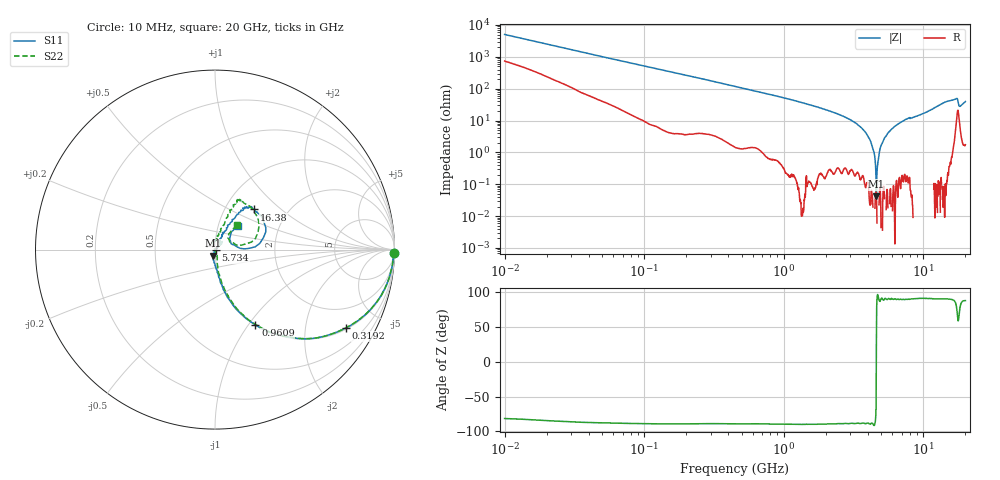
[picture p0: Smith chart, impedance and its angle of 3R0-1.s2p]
!Keysight Technologies,P5008B,MY61100088,A.16.20.02
!Date: Monday, May 27, 2024 14:41:35
!Correction: S11(C* 2-Port  )
!S21(C* 2-Port  )
!S12(C* 2-Port  )
!S22(C* 2-Port  )
!S2P File: Measurements: S11, S21, S12, S22:Log Frequency Sweep
# Hz S  dB  R 50
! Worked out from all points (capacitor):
!   1601 points, 10 MHz to 20 GHz, reference 50 ohm
!   read as one part in series: C = 3.2 pF near 10.39 MHz
!   lowest |Z| = 41.9 mohm at 4.608 GHz (marker M1)
!   series resonance near 4.605 GHz, so ESL is about 370 pH
!   S11 on the Smith chart (normalised r, x): 10 MHz: open; 319.2 MHz: 1.05, -3.30; 960.9 MHz: 1.00, -1.08; 5.734 GHz: 1.01, -0.00; 16.38 GHz: 1.37, +0.68; 20 GHz: 1.24, +0.34
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1e7  -0.01 -1.1  -34.07 80.4  -34.08 80.5  -0.03 -1.1
3.555162e7  -0.05 -4.0  -23.05 82.9  -23.05 82.9  -0.06 -4.0
1.263918e8  -0.29 -13.6  -12.63 75.6  -12.65 75.6  -0.28 -13.6
3.191771e8  -1.41 -31.0  -5.81 57.9  -5.82 57.9  -1.42 -30.9
4.472136e8  -2.40 -40.2  -3.87 49.2  -3.88 49.2  -2.39 -40.1
9.609065e8  -6.44 -61.8  -1.15 27.9  -1.16 27.9  -6.43 -61.5
1.589917e9  -10.71 -74.1  -0.38 16.1  -0.39 16.1  -10.66 -73.0
2.976524e9  -17.95 -83.9  -0.06 5.1  -0.07 5.1  -18.06 -81.1
4.608065e9  -29.07 -106.3  0.01 -1.9  -0.00 -1.9  -29.52 -71.0
5.28871e9  -37.50 -110.6  0.01 -4.1  0.00 -4.1  -37.01 -71.9
5.652411e9  -50.63 -65.1  0.02 -5.1  0.01 -5.1  -49.93 -92.1
5.733545e9  -45.82 -24.3  0.02 -5.4  0.01 -5.4  -53.95 -90.9
5.899321e9  -42.70 41.9  0.03 -5.9  0.01 -5.9  -45.68 124.1
6.098795e9  -36.17 30.6  0.03 -6.4  0.02 -6.4  -40.78 106.8
6.365204e9  -33.20 40.9  0.03 -7.1  0.01 -7.1  -35.88 102.6
7.340179e9  -26.11 43.9  0.02 -9.7  0.01 -9.7  -27.46 101.9
9.30816e9  -26.63 58.1  0.04 -14.4  0.03 -14.4  -26.32 90.0
1.367661e10  -12.48 56.8  -0.18 -25.6  -0.19 -25.6  -12.54 68.7
1.638242e10  -10.10 45.7  -0.48 -32.3  -0.48 -32.3  -10.24 63.1
1.717946e10  -9.90 34.4  -0.99 -35.1  -1.00 -35.1  -10.24 48.0
1.862442e10  -20.13 32.4  -0.28 -29.6  -0.29 -29.6  -20.36 41.8
2e10  -14.69 46.0  -0.24 -35.9  -0.25 -35.9  -14.55 48.1
